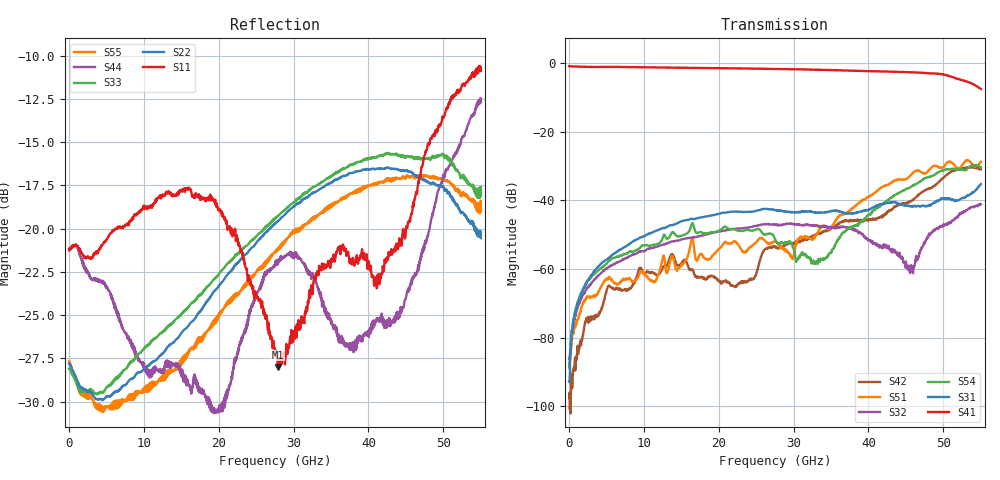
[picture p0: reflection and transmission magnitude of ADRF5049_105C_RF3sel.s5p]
! Device  : ADRF5049
! Description: Silicon SP4T Switch Non-Reflective
! Frequency:  9kHz -  45 GHz
! Ports:
!  RFC = Port 1
!  RF1 = Port 2
!  RF2 = Port 3
!	 RF3 = Port 4
!  RF4 = Port 5
! VSS  =  +3.30 Volts
! VDD  =  -3.30 Volts
! EN  =  0.00 Volts
! LS  =  0.00 Volts
! V1  =  0.00 Volts
! V2  =  3.30 Volts
! Data:  Data was collected using an calibrated 4 port network analyzer.
! Notes: Analog Devices supplies this data as a sample of measured data
!  for this product.  Your particular data for this product may vary.
!  Data was taken at 105 degrees C.
!  Analog Devices reserves the right to change this data at anytime.
# hz S db R 50
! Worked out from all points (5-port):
!   1100 points, 50 MHz to 55 GHz, reference 50 ohm
!   strongest paths, dB at 50 MHz, 13.8 GHz, 27.55 GHz, 41.3 GHz, 55 GHz:
!     S41: -0.9, -1.3, -1.7, -2.4, -7.5
!     S31: -92.8, -47.2, -42.8, -41.3, -35.2
!     S54: -87.6, -49.3, -51.5, -42.0, -30.4
!     S32: -86.1, -51.9, -47.0, -53.3, -41.2
!     S51: -88.1, -56.2, -51.8, -37.0, -28.7
!     S42: -97.5, -55.6, -53.5, -45.0, -30.9
!   lowest |S11| = -28.0 dB at 27.9 GHz (marker M1), VSWR 1.08, Z = 52.4 - j3.28 ohm
!   |S11| at or under -10 dB: start of sweep to end of sweep
